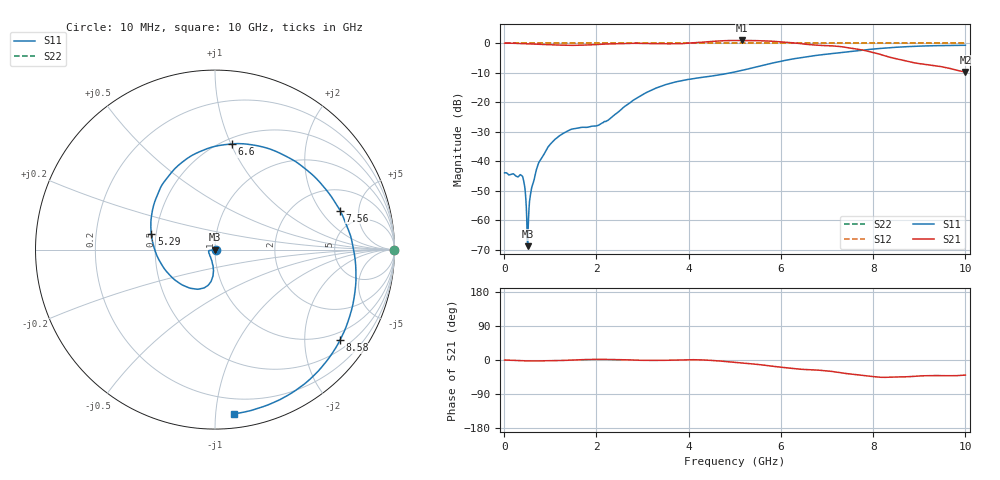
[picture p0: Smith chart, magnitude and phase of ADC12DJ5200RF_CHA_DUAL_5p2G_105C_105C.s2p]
! Texas Instruments, Inc.
! ADC12DJ5200RF - CH A S-Parameters (Dual Ch Mode, Fs = 5.2 GSPS, 105 degC case, 105 degC juntion)
! Port 1 represents the 100-ohm differenal input, Port 2 the digital output
! freq  dbS11  angS11  dbS21 angS21 dbS12 angS12 dbS22 angS22
# HZ S DB R 100
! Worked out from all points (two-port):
!   1000 points, 10 MHz to 10 GHz, reference 100 ohm
!   highest |S21| = 0.93 dB at 5.15 GHz (marker M1); lowest = -9.8 dB at 10 GHz (marker M2)
!   |S21| within 3 dB of the highest: start of sweep to 7.678 GHz
!   lowest |S11| = -68.9 dB at 510 MHz (marker M3), VSWR 1.00, Z = 100 - j0.0713 ohm
!   |S11| at or under -10 dB: start of sweep to 4.932 GHz
!   |S22| runs from 0.0 to 0.0 dB; largest |S21 - S12| = 0.78
!   S11 on the Smith chart (normalised r, x): 10 MHz: 1.01, -0.00; 5.29 GHz: 0.47, +0.10; 6.6 GHz: 0.55, +1.01; 7.56 GHz: 3.35, +3.13; 8.58 GHz: 0.75, -2.91; 10 GHz: 0.09, -1.12
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1e7  -43.98 -7.6  0.00 -0.1  0.00 0.0  0.00 0.0
3.8e8  -44.92 -10.5  -0.10 -1.9  0.00 0.0  0.00 0.0
4.3e8  -47.24 -0.5  -0.14 -2.1  0.00 0.0  0.00 0.0
4.7e8  -52.81 6.8  -0.17 -2.2  0.00 0.0  0.00 0.0
5.1e8  -68.87 -81.6  -0.19 -2.3  0.00 0.0  0.00 0.0
7.1e8  -42.37 -157.4  -0.35 -2.4  0.00 0.0  0.00 0.0
9.4e8  -35.52 -169.1  -0.50 -2.2  0.00 0.0  0.00 0.0
1.26e9  -30.80 -171.7  -0.67 -1.2  0.00 0.0  0.00 0.0
1.68e9  -28.56 -163.4  -0.67 0.8  0.00 0.0  0.00 0.0
2.24e9  -26.25 -119.8  -0.27 1.4  0.00 0.0  0.00 0.0
3.34e9  -14.98 -96.9  -0.18 -1.1  0.00 0.0  0.00 0.0
4.24e9  -11.72 -125.9  0.29 0.4  0.00 0.0  0.00 0.0
5.01e9  -9.74 -174.4  0.91 -6.4  0.00 0.0  0.00 0.0
5.15e9  -9.25 175.6  0.93 -7.8  0.00 0.0  0.00 0.0
5.29e9  -8.74 165.9  0.88 -9.3  0.00 0.0  0.00 0.0
5.9e9  -6.49 126.2  0.57 -17.6  0.00 0.0  0.00 0.0
6.6e9  -4.49 81.1  -0.43 -25.4  0.00 0.0  0.00 0.0
6.67e9  -4.33 76.5  -0.54 -26.0  0.00 0.0  0.00 0.0
7.56e9  -2.73 17.4  -1.79 -37.7  0.00 0.0  0.00 0.0
8.34e9  -1.56 -25.8  -4.68 -45.5  0.00 0.0  0.00 0.0
8.58e9  -1.31 -35.9  -5.53 -44.6  0.00 0.0  0.00 0.0
1e10  -0.71 -83.2  -9.76 -39.8  0.00 0.0  0.00 0.0
